(* Logix 5000 AddOnInstructionDefinition export AKD_Motion_Status; software revision 19.01 *)

TYPE AKD_Status :   // All connections to the drive ethernet module are established and data is successfully transferring.
STRUCT
   Profile_In_Progress : BOOL;   // Profile Move In Progress
   Block_In_Execution : BOOL;   // Block In Execution
   On_Target_Position : BOOL;   // On Target Position (1=Current Position Equals Last Target Position)
   General_Fault : BOOL;   // General Fault
   Current_Direction : BOOL;   // Current Motor Direction (0=Reverse, 1=Forward)
   Home_Level : BOOL;   // Level of Home Input
   Reg_Level : BOOL;   // Level of Registration Input
   Enable : BOOL;   // State of Enable Output
   Fault_Input_Fault : BOOL;   // Fault Input Active
   Fwd_Limit : BOOL;   // Forward Input Active
   Rev_Limit : BOOL;   // Reverse Input Active
   Positive_Limit : BOOL;   // Positive Software Limit Exceeded
   Negative_Limit : BOOL;   // Negative Software Limit Exceeded
   FE_Fault : BOOL;   // Following Error Fault
   Block_Fault : BOOL;   // Block Execution Fault
   Load_Complete : BOOL;   // Command Message Successfully Loaded
END_STRUCT
END_TYPE

TYPE AKD_Control :   // Send Explicit Message
STRUCT
   Load_Data_Start_Profile : BOOL;   // Load Command Data / Start Profile Move
   Start_Block : BOOL;   // Execute Command block or block chain
   Incremental : BOOL;   // Incremental Position (0=Absolute, 1=Incremental)
   Direction : BOOL;   // Direction in Velocity Mode (0=Reverse, 1=Forward)
   Smooth_Stop : BOOL;   // Smooth / Controlled Stop w/ Deceleration
   Hard_Stop : BOOL;   // Hard / Immediate Stop
   Reg_Arm : BOOL;   // Arm the Registration Input
   Enable : BOOL;   // Enable Output
END_STRUCT
END_TYPE

TYPE AKD_Axis :   // Axis Data:
STRUCT
   Control : AKD_Control;   // Control bits to send to the drive
   Status : AKD_Status;   // Status bits received from the drive
   Input : AB:ETHERNET_MODULE_SINT_64Bytes:I:0;   // Data from the drive
   Output : AB:ETHERNET_MODULE_SINT_64Bytes:O:0;   // Data to the drive
   ResponseMsgType : SINT;   // Response type contained in latest IO response from drive. Used to check for errors
   CommandTimeout : INT;   // Time to allow for command response from drive. Dependent on scan rate and communicaiton rate
   PositionFeedback : DINT;   // Actual Position Value
   VelocityFeedback : DINT;   // Actual Velocity Value
END_STRUCT
END_TYPE

ADD_ON_INSTRUCTION AKD_Motion_Status   (* revision 2.0 *)
// Revision note:
// DRV.MOTIONSTAT upper status bits changed after FW 1.13.  Changed AOI output names to reflect changes and conform to FW 1.15. Reordered Target Position Crossed and In Target Position Window on the outputs so they are displayed in the same order as DRV.MOTIONSTAT in WB Help.
VAR_IN_OUT
   Axis : AKD_Axis; {required}
END_VAR
VAR_OUTPUT
   Motion_Task_Active : BOOL; {access Read Only, visible}
   Home_Position_Found : BOOL; {access Read Only, visible}
   Homing_Complete : BOOL; {access Read Only, visible}
   Homing_Active : BOOL; {access Read Only, visible}
   Homing_Error : BOOL; {access Read Only, visible}
   Gearing_Slave_Synchronized : BOOL; {access Read Only, visible}
   Gearing_Mode_Active : BOOL; {access Read Only, visible}
   ESTOP_In_Progress : BOOL; {access Read Only, visible}
   ESTOP_Error : BOOL; {access Read Only, visible}
   Service_Motion_Active : BOOL; {access Read Only, visible}
   Motion_Task_Activation_Failed : BOOL; {access Read Only, visible}
   Motion_Task_Target_Position_Reached : BOOL; {access Read Only, visible}
   Motion_Task_Target_Velocity_Reached : BOOL; {access Read Only, visible}
   Motion_Task_Exception : BOOL; {access Read Only, visible}
   Motion_Task_Target_Position_Crossed : BOOL; {access Read Only, visible}
   Motion_Task_In_Target_Position_Window : BOOL; {access Read Only, visible}
   In_Homing_Target_Position_Window : BOOL; {access Read Only, visible}
   Cogging_Comp_Teach_Move_Active : BOOL; {access Read Only, visible}
END_VAR

ROUTINE Logic   (* ladder *)
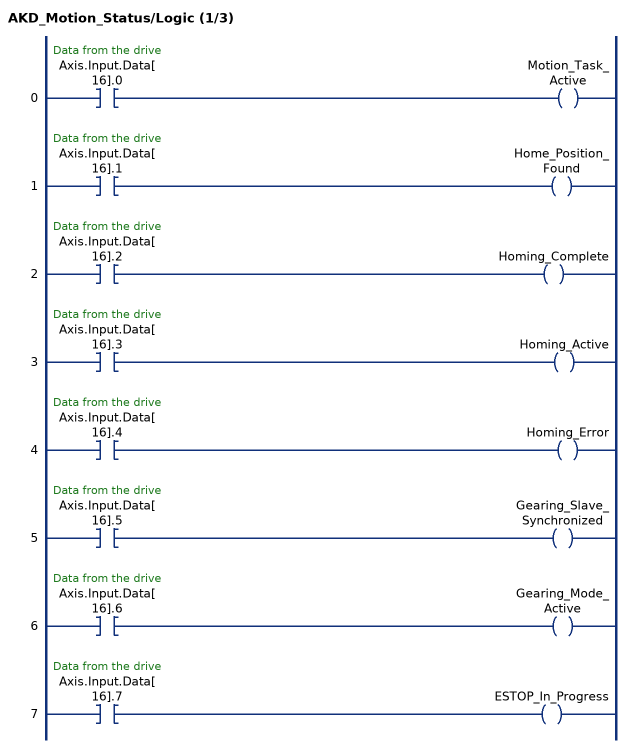
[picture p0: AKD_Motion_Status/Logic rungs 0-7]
   0: XIC(Axis.Input.Data[16].0)OTE(Motion_Task_Active);
   1: XIC(Axis.Input.Data[16].1)OTE(Home_Position_Found);
   2: XIC(Axis.Input.Data[16].2)OTE(Homing_Complete);
   3: XIC(Axis.Input.Data[16].3)OTE(Homing_Active);
   4: XIC(Axis.Input.Data[16].4)OTE(Homing_Error);
   5: XIC(Axis.Input.Data[16].5)OTE(Gearing_Slave_Synchronized);
   6: XIC(Axis.Input.Data[16].6)OTE(Gearing_Mode_Active);
   7: XIC(Axis.Input.Data[16].7)OTE(ESTOP_In_Progress);
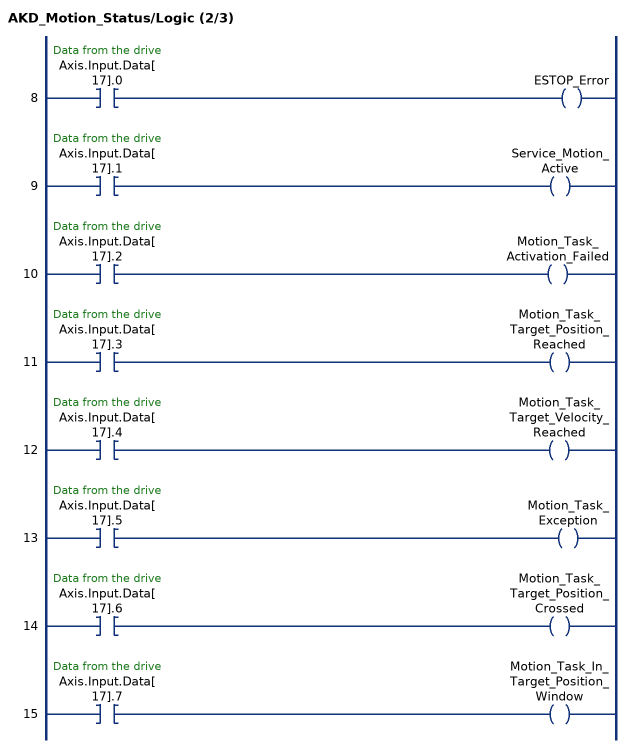
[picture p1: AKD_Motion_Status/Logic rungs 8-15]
   8: XIC(Axis.Input.Data[17].0)OTE(ESTOP_Error);
   9: XIC(Axis.Input.Data[17].1)OTE(Service_Motion_Active);
   10: XIC(Axis.Input.Data[17].2)OTE(Motion_Task_Activation_Failed);
   11: XIC(Axis.Input.Data[17].3)OTE(Motion_Task_Target_Position_Reached);
   12: XIC(Axis.Input.Data[17].4)OTE(Motion_Task_Target_Velocity_Reached);
   13: XIC(Axis.Input.Data[17].5)OTE(Motion_Task_Exception);
   14: XIC(Axis.Input.Data[17].6)OTE(Motion_Task_Target_Position_Crossed);
   15: XIC(Axis.Input.Data[17].7)OTE(Motion_Task_In_Target_Position_Window);
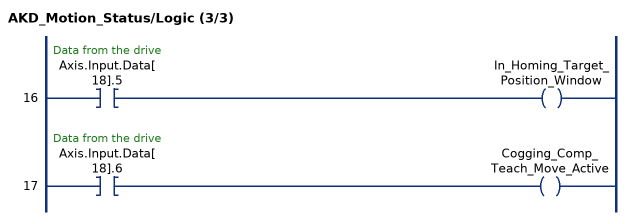
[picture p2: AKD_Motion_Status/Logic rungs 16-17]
   16: XIC(Axis.Input.Data[18].5)OTE(In_Homing_Target_Position_Window);
   17: XIC(Axis.Input.Data[18].6)OTE(Cogging_Comp_Teach_Move_Active);
END_ROUTINE
END_ADD_ON_INSTRUCTION
